(* Logix 5000 AddOnInstructionDefinition export YAI_Assy_166_101_EIP_Hz; software revision 17.00 *)

ADD_ON_INSTRUCTION YAI_Assy_166_101_EIP_Hz   (* revision 1.0, vendor Yaskawa America, Inc. *)
// YAI Assembly 166 and 101
// Help:
// This add-on instruction is for use with input assemblie 166 and output assemblies 116.
// Node_Input_Assy is defined as the node's input assembly integer array.
// Node_Output_Assy is defined as the node's output assembly integer array.
// Torque limit/reference, torque compensation and torque output variables are only available with A1000.
VAR_IN_OUT
   Node_Input_Assy : AB:ETHERNET_MODULE_INT_44Bytes:I:0; {required}   // Input assembly words
   Node_Output_Assy : AB:ETHERNET_MODULE_INT_8Bytes:O:0; {required}   // Output assembly words
END_VAR
VAR_INPUT
   RunFwd : BOOL; {visible}   // Forward run command
   RunRev : BOOL; {visible}   // Reverse run command
   FaultReset : BOOL; {visible}   // Fault reset command
   Freq_Ref : REAL; {visible}   // Frequency reference command in Hz (xx.xx resolution)
   Net_Ref : BOOL;   // Network reference control bit
   Net_Control : BOOL;   // Network start/stop control bit
END_VAR
VAR_OUTPUT
   Running : BOOL; {visible}   // Drive running forward status bit
   ZSP : BOOL; {visible}   // Drive zero speed status bit
   RunningRev : BOOL; {visible}   // Drive running reverse status bit
   Reset : BOOL; {visible}   // Drive reset command status bit
   At_Speed : BOOL; {visible}   // Drive at commanded speed status bit
   Ready : BOOL; {visible}   // Drive ready status bit
   Alarm : BOOL; {visible}   // Drive alarm status bit
   Faulted : BOOL; {visible}   // Drive faulted status bit
   OPE : BOOL;   // OPE alarm/fault present
   UV : BOOL;   // Drive in UV (undervoltage) state status bit
   NetCtrlStatus : BOOL; {visible}   // Drive network run source status bit (1 = source coming from network)
   MFO_1_Status : BOOL; {visible}   // Drive multi-function output 1 (M1-M2 for A/P1000, MA/MB/MC for V1000) status
   MFO_2_Status : BOOL; {visible}   // Drive multi-function output 1 (M3-M4 for A/P1000, P1 for V1000) status
   MFO_3_Status : BOOL; {visible}   // Drive multi-function output 1 (M5-M6 for A/P1000, P2 for V1000) status
   ZSV : BOOL; {visible}   // Drive zero servo completed status bit
   Motor_Speed : REAL; {visible}   // Motor speed in Hz (xx.xx resolution)
   Torque_Actual : REAL; {visible}   // Drive torque output in % (xxx.x resolution)
   PG_Count : INT;   // Encoder feedback count
   Freq_Cmd : REAL; {visible}   // Commanded frequency in Hz (xx.xx resolution)
   Output_Freq : REAL; {visible}   // Drive output frequency in Hz (xx.xx resolution)
   Output_Current : REAL; {visible}   // Drive output current in A (xxx.x resolution)
   Analog_Input_1_Level : REAL;   // Analog input 1 level in % (xxx.x resolution)
   DC_Bus_Volt : INT; {visible}   // DC bus voltage in Vdc (xxx resolution)
   Error_Code : INT;   // Custom input/output error code. Refer to custom error bit to determine which parameter error is pertaining to.
   Custom_In_1 : INT; {visible}   // Custom input 1 - F7-33
   Custom_In_2 : INT; {visible}   // Custom input 2 - F7-34
   Custom_In_3 : INT; {visible}   // Custom input 3 - F7-35
   Custom_In_4 : INT;   // Custom input 4 - F7-36
   Custom_In_5 : INT;   // Custom input 5 - F7-37
   Custom_In_6 : INT;   // Custom input 6 - F7-38
   Custom_In_7 : INT;   // Custom input 7 - F7-39
   Custom_In_8 : INT;   // Custom input 8 -F7-40
   Custom_In_9 : INT;   // Custom input 9 - F7-41
   Custom_In_10 : INT;   // Custom input 10 - F7-42
   Custom_In_1_Error : BOOL;   // Custom input 1 error bit
   Custom_In_2_Error : BOOL;   // Custom input 2 error bit
   Custom_In_3_Error : BOOL;   // Custom input 3 error bit
   Custom_In_4_Error : BOOL;   // Custom input 4 error bit
   Custom_In_5_Error : BOOL;   // Custom input 5 error bit
   Custom_In_6_Error : BOOL;   // Custom input 6 error bit
   Custom_In_7_Error : BOOL;   // Custom input 7 error bit
   Custom_In_8_Error : BOOL;   // Custom input 8 error bit
   Custom_In_9_Error : BOOL;   // Custom input 9 error bit
   Custom_In_10_Error : BOOL;   // Custom input 10 error bit
END_VAR
VAR_INPUT
   Motor_Rated_Torq : REAL;
   MFI_3 : BOOL;
   MFI_4 : BOOL;
   MFI_5 : BOOL;
   MFI_6 : BOOL;
   MFI_7 : BOOL;
   External_Fault : BOOL;
   MFI_8 : BOOL;
   MFO_1 : BOOL;
   MFO_2 : BOOL;
   MFO_3 : BOOL;
   Torq_Ref_Limit : REAL;
   Torq_Comp : REAL;
END_VAR
VAR
   FRef_Convert : DINT;
   FOut_Convert : REAL;
   FOut_Temp : REAL;
   TRef_Convert : INT;
   TComp_Convert : INT;
   TOut_Convert : REAL;
   TOut_Temp : REAL;
   IOut_Temp : REAL;
   IOut_Convert : REAL;
   AO1_Convert : INT;
   AO2_Convert : INT;
   Motor_Speed_Temp : REAL;
   Motor_Speed_Convert : REAL;
   Freq_Cmd_Temp : REAL;
   Freq_Cmd_Convert : REAL;
   AI1_Temp : REAL;
   AI1_Convert : REAL;
   Motor_Torq_Temp : REAL;
END_VAR

ROUTINE Logic   (* ladder *)
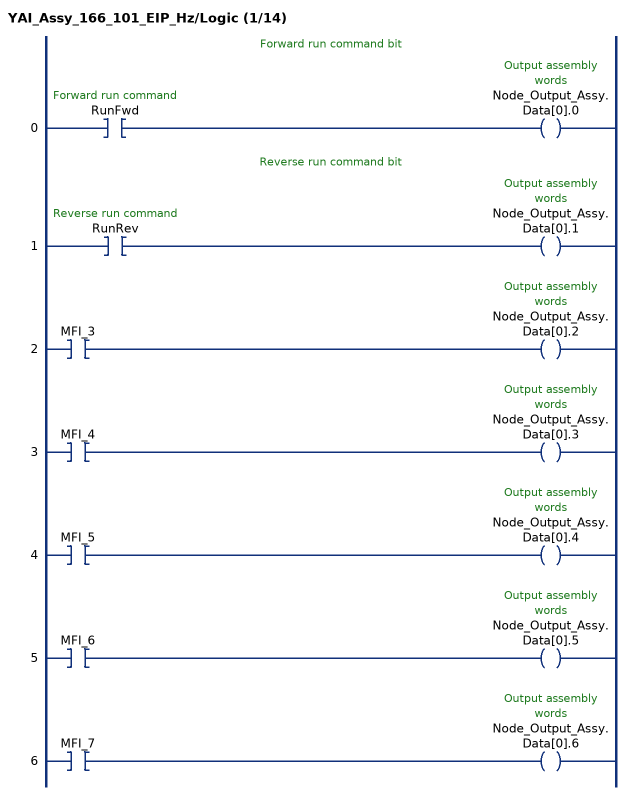
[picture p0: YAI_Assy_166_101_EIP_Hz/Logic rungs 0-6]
   // Forward run command bit
   0: XIC(RunFwd)OTE(Node_Output_Assy.Data[0].0);
   // Reverse run command bit
   1: XIC(RunRev)OTE(Node_Output_Assy.Data[0].1);
   2: XIC(MFI_3)OTE(Node_Output_Assy.Data[0].2);
   3: XIC(MFI_4)OTE(Node_Output_Assy.Data[0].3);
   4: XIC(MFI_5)OTE(Node_Output_Assy.Data[0].4);
   5: XIC(MFI_6)OTE(Node_Output_Assy.Data[0].5);
   6: XIC(MFI_7)OTE(Node_Output_Assy.Data[0].6);
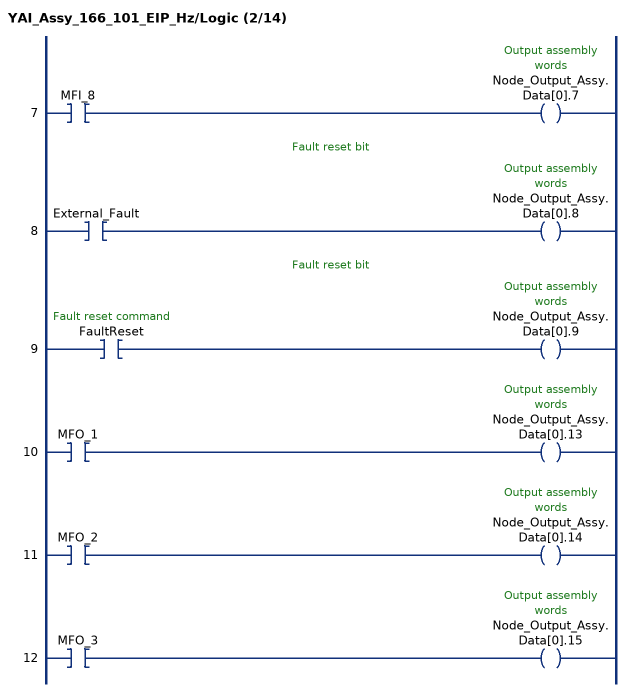
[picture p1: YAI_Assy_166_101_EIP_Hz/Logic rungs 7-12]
   7: XIC(MFI_8)OTE(Node_Output_Assy.Data[0].7);
   // Fault reset bit
   8: XIC(External_Fault)OTE(Node_Output_Assy.Data[0].8);
   // Fault reset bit
   9: XIC(FaultReset)OTE(Node_Output_Assy.Data[0].9);
   10: XIC(MFO_1)OTE(Node_Output_Assy.Data[0].13);
   11: XIC(MFO_2)OTE(Node_Output_Assy.Data[0].14);
   12: XIC(MFO_3)OTE(Node_Output_Assy.Data[0].15);
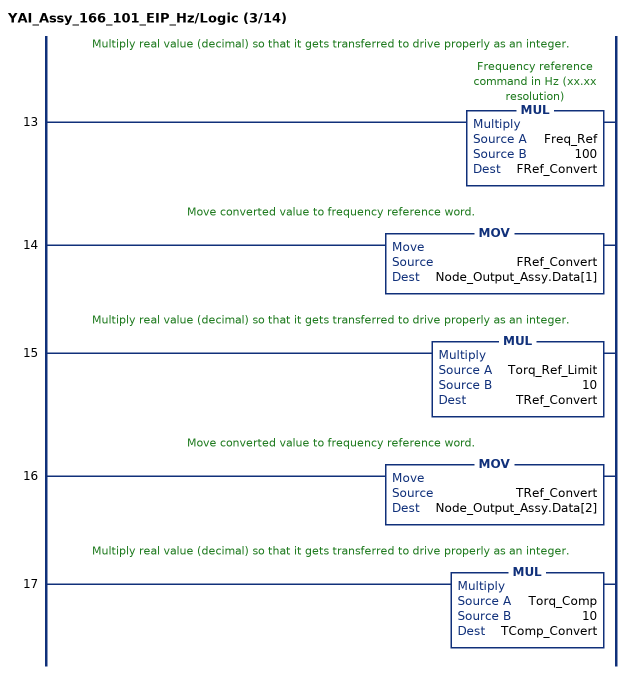
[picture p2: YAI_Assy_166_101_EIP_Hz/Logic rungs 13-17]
   // Multiply real value (decimal) so that it gets transferred to drive properly as an integer.
   13: MUL(Freq_Ref,100,FRef_Convert);
   // Move converted value to frequency reference word.
   14: MOV(FRef_Convert,Node_Output_Assy.Data[1]);
   // Multiply real value (decimal) so that it gets transferred to drive properly as an integer.
   15: MUL(Torq_Ref_Limit,10,TRef_Convert);
   // Move converted value to frequency reference word.
   16: MOV(TRef_Convert,Node_Output_Assy.Data[2]);
   // Multiply real value (decimal) so that it gets transferred to drive properly as an integer.
   17: MUL(Torq_Comp,10,TComp_Convert);
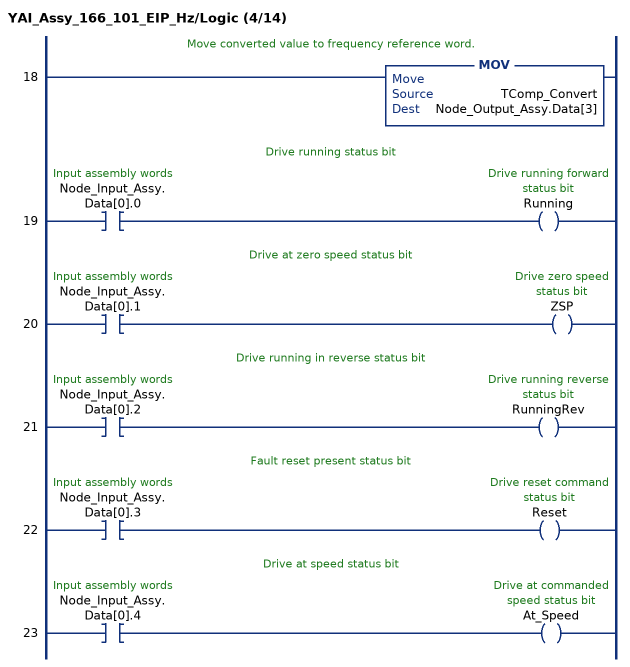
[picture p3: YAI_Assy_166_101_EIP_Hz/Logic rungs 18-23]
   // Move converted value to frequency reference word.
   18: MOV(TComp_Convert,Node_Output_Assy.Data[3]);
   // Drive running status bit
   19: XIC(Node_Input_Assy.Data[0].0)OTE(Running);
   // Drive at zero speed status bit
   20: XIC(Node_Input_Assy.Data[0].1)OTE(ZSP);
   // Drive running in reverse status bit
   21: XIC(Node_Input_Assy.Data[0].2)OTE(RunningRev);
   // Fault reset present status bit
   22: XIC(Node_Input_Assy.Data[0].3)OTE(Reset);
   // Drive at speed status bit
   23: XIC(Node_Input_Assy.Data[0].4)OTE(At_Speed);
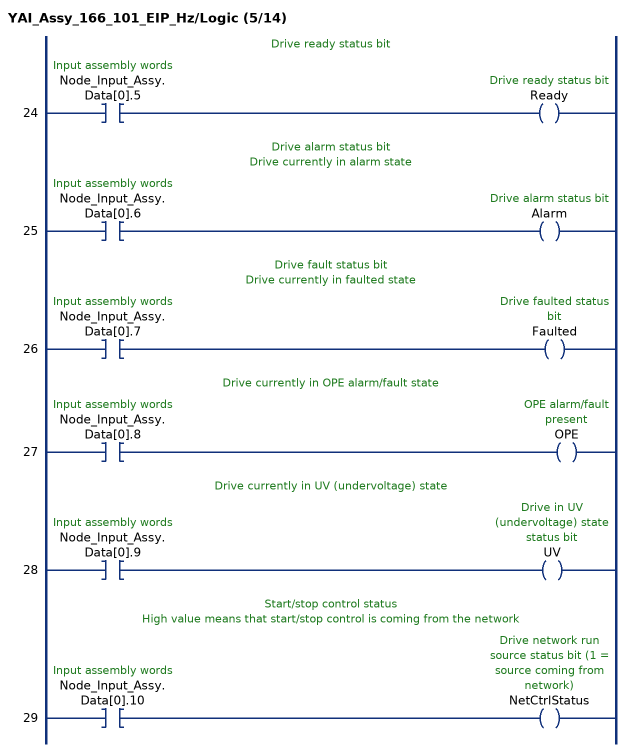
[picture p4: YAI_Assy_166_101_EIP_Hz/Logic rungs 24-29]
   // Drive ready status bit
   24: XIC(Node_Input_Assy.Data[0].5)OTE(Ready);
   // Drive alarm status bit
   // Drive currently in alarm state
   25: XIC(Node_Input_Assy.Data[0].6)OTE(Alarm);
   // Drive fault status bit
   // Drive currently in faulted state
   26: XIC(Node_Input_Assy.Data[0].7)OTE(Faulted);
   // Drive currently in OPE alarm/fault state
   27: XIC(Node_Input_Assy.Data[0].8)OTE(OPE);
   // Drive currently in UV (undervoltage) state
   28: XIC(Node_Input_Assy.Data[0].9)OTE(UV);
   // Start/stop control status
   // High value means that start/stop control is coming from the network
   29: XIC(Node_Input_Assy.Data[0].10)OTE(NetCtrlStatus);
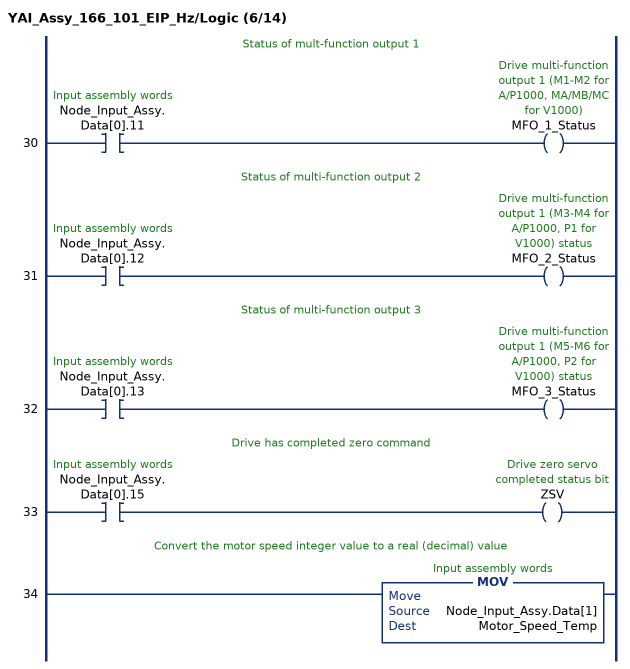
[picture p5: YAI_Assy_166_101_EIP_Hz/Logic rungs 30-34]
   // Status of mult-function output 1
   30: XIC(Node_Input_Assy.Data[0].11)OTE(MFO_1_Status);
   // Status of multi-function output 2
   31: XIC(Node_Input_Assy.Data[0].12)OTE(MFO_2_Status);
   // Status of multi-function output 3
   32: XIC(Node_Input_Assy.Data[0].13)OTE(MFO_3_Status);
   // Drive has completed zero command
   33: XIC(Node_Input_Assy.Data[0].15)OTE(ZSV);
   // Convert the motor speed integer value to a real (decimal) value
   34: MOV(Node_Input_Assy.Data[1],Motor_Speed_Temp);
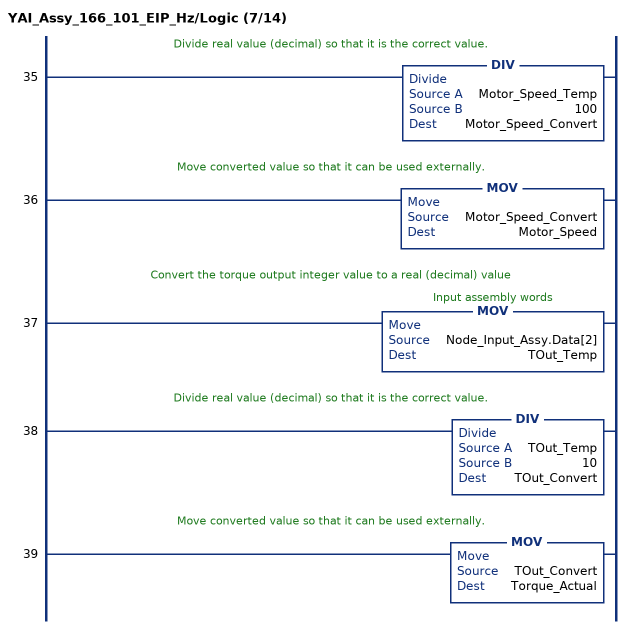
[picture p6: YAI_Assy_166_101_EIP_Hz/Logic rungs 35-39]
   // Divide real value (decimal) so that it is the correct value.
   35: DIV(Motor_Speed_Temp,100,Motor_Speed_Convert);
   // Move converted value so that it can be used externally.
   36: MOV(Motor_Speed_Convert,Motor_Speed);
   // Convert the torque output integer value to a real (decimal) value
   37: MOV(Node_Input_Assy.Data[2],TOut_Temp);
   // Divide real value (decimal) so that it is the correct value.
   38: DIV(TOut_Temp,10,TOut_Convert);
   // Move converted value so that it can be used externally.
   39: MOV(TOut_Convert,Torque_Actual);
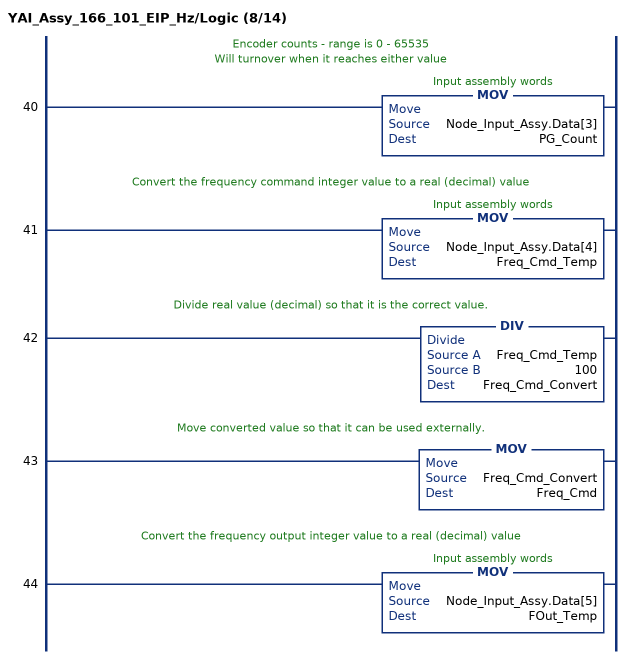
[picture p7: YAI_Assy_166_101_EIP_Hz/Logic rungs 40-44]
   // Encoder counts - range is 0 - 65535
   // Will turnover when it reaches either value
   40: MOV(Node_Input_Assy.Data[3],PG_Count);
   // Convert the frequency command integer value to a real (decimal) value
   41: MOV(Node_Input_Assy.Data[4],Freq_Cmd_Temp);
   // Divide real value (decimal) so that it is the correct value.
   42: DIV(Freq_Cmd_Temp,100,Freq_Cmd_Convert);
   // Move converted value so that it can be used externally.
   43: MOV(Freq_Cmd_Convert,Freq_Cmd);
   // Convert the frequency output integer value to a real (decimal) value
   44: MOV(Node_Input_Assy.Data[5],FOut_Temp);
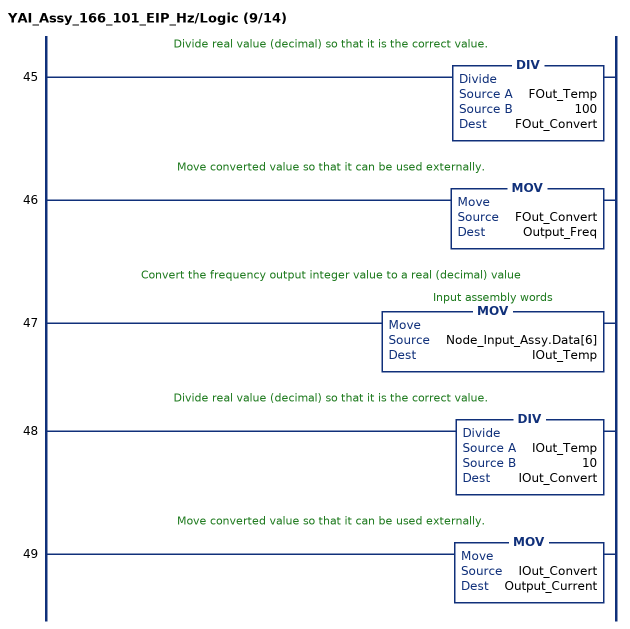
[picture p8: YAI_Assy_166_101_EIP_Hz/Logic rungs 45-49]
   // Divide real value (decimal) so that it is the correct value.
   45: DIV(FOut_Temp,100,FOut_Convert);
   // Move converted value so that it can be used externally.
   46: MOV(FOut_Convert,Output_Freq);
   // Convert the frequency output integer value to a real (decimal) value
   47: MOV(Node_Input_Assy.Data[6],IOut_Temp);
   // Divide real value (decimal) so that it is the correct value.
   48: DIV(IOut_Temp,10,IOut_Convert);
   // Move converted value so that it can be used externally.
   49: MOV(IOut_Convert,Output_Current);
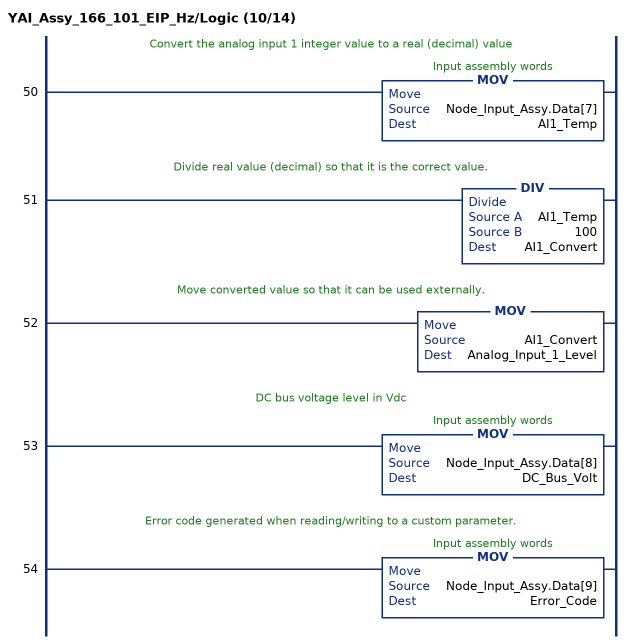
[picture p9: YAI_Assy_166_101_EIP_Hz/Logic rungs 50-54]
   // Convert the analog input 1 integer value to a real (decimal) value
   50: MOV(Node_Input_Assy.Data[7],AI1_Temp);
   // Divide real value (decimal) so that it is the correct value.
   51: DIV(AI1_Temp,100,AI1_Convert);
   // Move converted value so that it can be used externally.
   52: MOV(AI1_Convert,Analog_Input_1_Level);
   // DC bus voltage level in Vdc
   53: MOV(Node_Input_Assy.Data[8],DC_Bus_Volt);
   // Error code generated when reading/writing to a custom parameter.
   54: MOV(Node_Input_Assy.Data[9],Error_Code);
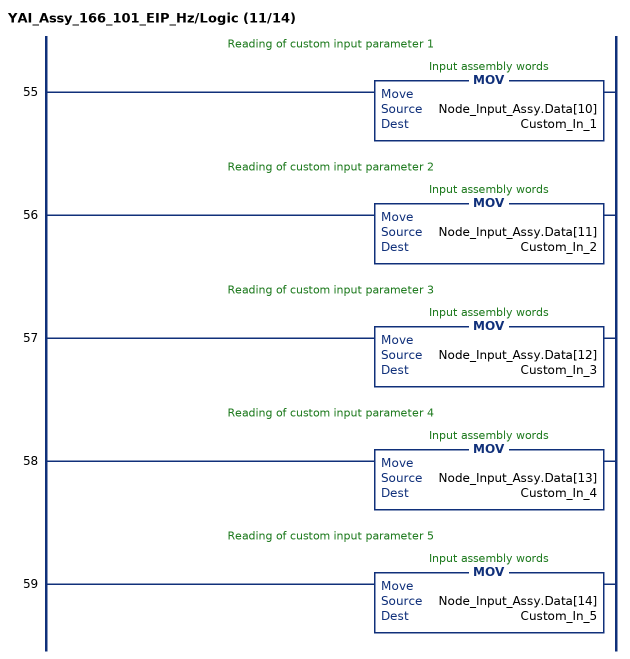
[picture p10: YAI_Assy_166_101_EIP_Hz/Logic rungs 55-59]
   // Reading of custom input parameter 1
   55: MOV(Node_Input_Assy.Data[10],Custom_In_1);
   // Reading of custom input parameter 2
   56: MOV(Node_Input_Assy.Data[11],Custom_In_2);
   // Reading of custom input parameter 3
   57: MOV(Node_Input_Assy.Data[12],Custom_In_3);
   // Reading of custom input parameter 4
   58: MOV(Node_Input_Assy.Data[13],Custom_In_4);
   // Reading of custom input parameter 5
   59: MOV(Node_Input_Assy.Data[14],Custom_In_5);
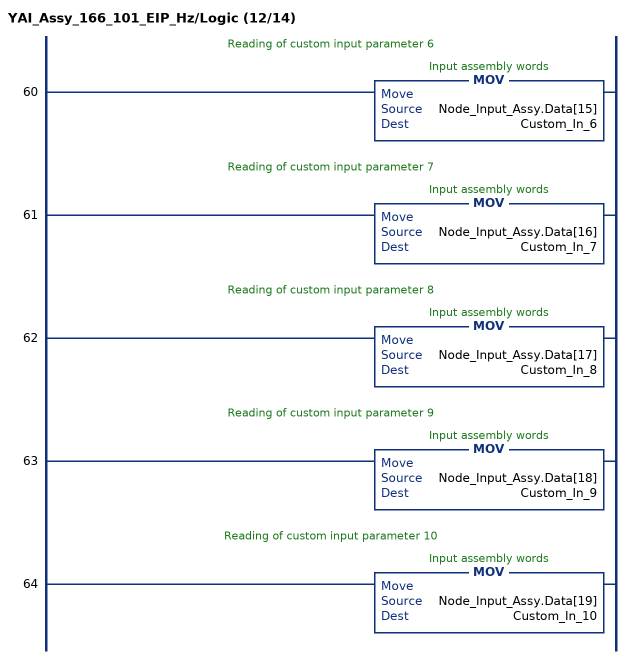
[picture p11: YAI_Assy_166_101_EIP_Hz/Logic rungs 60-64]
   // Reading of custom input parameter 6
   60: MOV(Node_Input_Assy.Data[15],Custom_In_6);
   // Reading of custom input parameter 7
   61: MOV(Node_Input_Assy.Data[16],Custom_In_7);
   // Reading of custom input parameter 8
   62: MOV(Node_Input_Assy.Data[17],Custom_In_8);
   // Reading of custom input parameter 9
   63: MOV(Node_Input_Assy.Data[18],Custom_In_9);
   // Reading of custom input parameter 10
   64: MOV(Node_Input_Assy.Data[19],Custom_In_10);
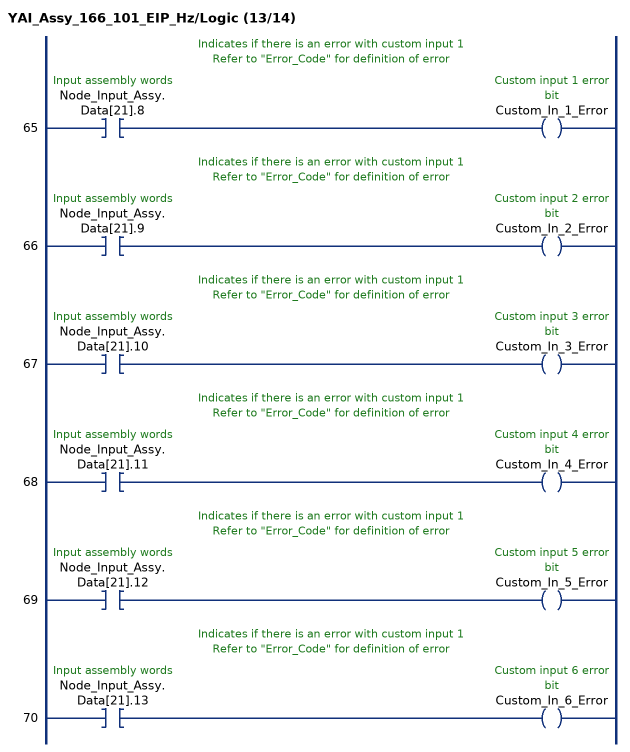
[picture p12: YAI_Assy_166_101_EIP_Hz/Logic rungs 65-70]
   // Indicates if there is an error with custom input 1
   // Refer to "Error_Code" for definition of error
   65: XIC(Node_Input_Assy.Data[21].8)OTE(Custom_In_1_Error);
   // Indicates if there is an error with custom input 1
   // Refer to "Error_Code" for definition of error
   66: XIC(Node_Input_Assy.Data[21].9)OTE(Custom_In_2_Error);
   // Indicates if there is an error with custom input 1
   // Refer to "Error_Code" for definition of error
   67: XIC(Node_Input_Assy.Data[21].10)OTE(Custom_In_3_Error);
   // Indicates if there is an error with custom input 1
   // Refer to "Error_Code" for definition of error
   68: XIC(Node_Input_Assy.Data[21].11)OTE(Custom_In_4_Error);
   // Indicates if there is an error with custom input 1
   // Refer to "Error_Code" for definition of error
   69: XIC(Node_Input_Assy.Data[21].12)OTE(Custom_In_5_Error);
   // Indicates if there is an error with custom input 1
   // Refer to "Error_Code" for definition of error
   70: XIC(Node_Input_Assy.Data[21].13)OTE(Custom_In_6_Error);
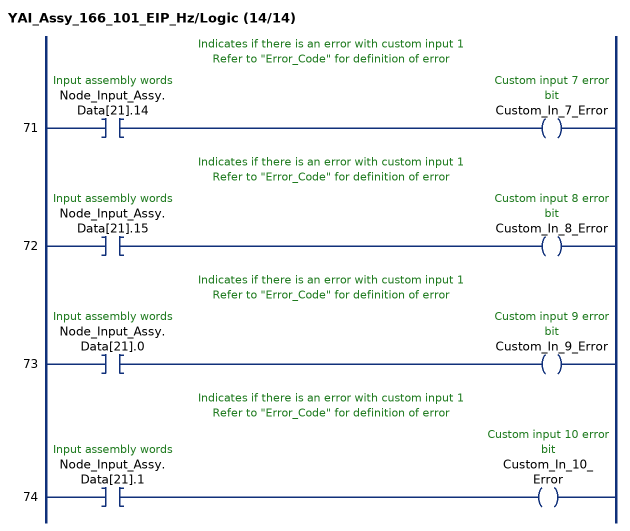
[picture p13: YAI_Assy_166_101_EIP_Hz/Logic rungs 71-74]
   // Indicates if there is an error with custom input 1
   // Refer to "Error_Code" for definition of error
   71: XIC(Node_Input_Assy.Data[21].14)OTE(Custom_In_7_Error);
   // Indicates if there is an error with custom input 1
   // Refer to "Error_Code" for definition of error
   72: XIC(Node_Input_Assy.Data[21].15)OTE(Custom_In_8_Error);
   // Indicates if there is an error with custom input 1
   // Refer to "Error_Code" for definition of error
   73: XIC(Node_Input_Assy.Data[21].0)OTE(Custom_In_9_Error);
   // Indicates if there is an error with custom input 1
   // Refer to "Error_Code" for definition of error
   74: XIC(Node_Input_Assy.Data[21].1)OTE(Custom_In_10_Error);
END_ROUTINE
END_ADD_ON_INSTRUCTION
